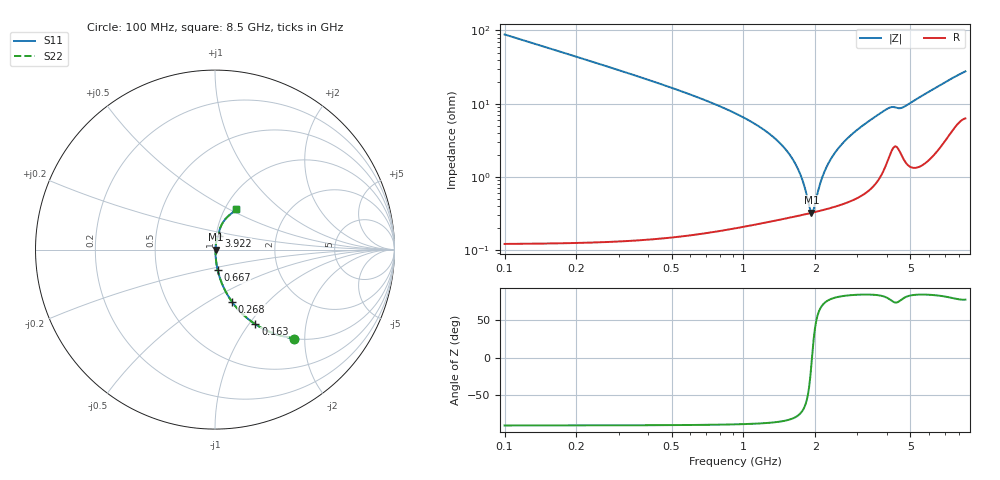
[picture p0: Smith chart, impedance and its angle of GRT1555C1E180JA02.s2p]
!Murata Part Number: GRT1555C1E180JA02
!These Parameters are Measured in Series Mode Connection
!Data Generated on Jun 19, 2026
!  o--ll--o
!Port1  Port2
!  o------o
!Operation Temp=25[degC], DC Bias Voltage=0[V]
!Freq. Start=100[MHz] Stop=9[GHz] 401[Steps]
# Hz S RI R 50
!Freq.(Hz) S11(Real) S11(Imag) S21(Real) S21(Imag) S12(Real) S12(Imag) S22(Real) S22(Imag)
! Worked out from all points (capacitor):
!   401 points, 100 MHz to 8.5 GHz, reference 50 ohm
!   read as one part in series: C = 18 pF near 142 MHz
!   lowest |Z| = 326 mohm at 1.927 GHz (marker M1)
!   series resonance near 1.937 GHz, so ESL is about 370 pH
!   S11 on the Smith chart (normalised r, x): 100 MHz: 1.00, -1.76; 163 MHz: 1.00, -1.08; 268 MHz: 1.00, -0.65; 667 MHz: 1.00, -0.23; 3.922 GHz: 1.03, +0.16; 8.5 GHz: 1.13, +0.54
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1e8  0.4375 -0.4954  0.5625 0.4954  0.5625 0.4954  0.4375 -0.4954
1.63e8  0.2254 -0.4167  0.7746 0.4167  0.7746 0.4167  0.2254 -0.4167
2.68e8  0.0957 -0.2922  0.9043 0.2922  0.9043 0.2922  0.0957 -0.2922
4.36e8  0.037 -0.185  0.963 0.185  0.963 0.185  0.037 -0.185
6.67e8  0.015 -0.1148  0.985 0.1148  0.985 0.1148  0.015 -0.1148
1.234e9  0.00416 -0.0424  0.9958 0.0424  0.9958 0.0424  0.00416 -0.0424
1.507e9  0.00323 -0.0231  0.9968 0.0231  0.9968 0.0231  0.00323 -0.0231
1.717e9  0.00307 -0.0111  0.9969 0.0111  0.9969 0.0111  0.00307 -0.0111
1.885e9  0.00316 -0.0025  0.9968 0.0025  0.9968 0.0025  0.00316 -0.0025
1.927e9  0.00321 -0.000476  0.9968 0.000476  0.9968 0.000476  0.00321 -0.000476
1.969e9  0.00327 0.00151  0.9967 -0.00151  0.9967 -0.00151  0.00327 0.00151
2.074e9  0.00344 0.00632  0.9966 -0.00632  0.9966 -0.00632  0.00344 0.00632
2.158e9  0.00361 0.01  0.9964 -0.01  0.9964 -0.01  0.00361 0.01
2.305e9  0.00399 0.0163  0.996 -0.0163  0.996 -0.0163  0.00399 0.0163
2.557e9  0.00483 0.0264  0.9952 -0.0264  0.9952 -0.0264  0.00483 0.0264
2.914e9  0.00649 0.0401  0.9935 -0.0401  0.9935 -0.0401  0.00649 0.0401
3.922e9  0.0196 0.0781  0.9804 -0.0781  0.9804 -0.0781  0.0196 0.0781
4.3e9  0.032 0.0806  0.968 -0.0806  0.968 -0.0806  0.032 0.0806
4.615e9  0.0257 0.0822  0.9743 -0.0822  0.9743 -0.0822  0.0257 0.0822
5.707e9  0.0312 0.1264  0.9688 -0.1264  0.9688 -0.1264  0.0312 0.1264
7.114e9  0.0674 0.1806  0.9326 -0.1806  0.9326 -0.1806  0.0674 0.1806
8.5e9  0.1157 0.2237  0.8843 -0.2237  0.8843 -0.2237  0.1157 0.2237
